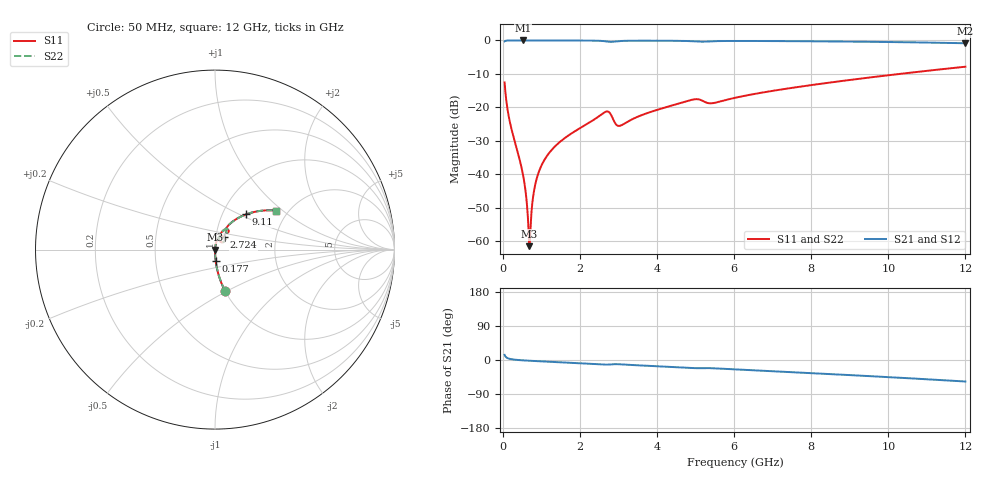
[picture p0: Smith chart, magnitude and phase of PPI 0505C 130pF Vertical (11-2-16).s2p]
# GHz S MA R 50
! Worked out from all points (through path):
!   1601 points, 50 MHz to 12 GHz, reference 50 ohm
!   highest |S21| = -0.01 dB at 528 MHz (marker M1); lowest = -0.8 dB at 12 GHz (marker M2)
!   group delay of S21, straight-line fit = 13.2 ps
!   lowest |S11| = -61.4 dB at 692.3 MHz (marker M3), VSWR 1.00, Z = 50.1 - j0.0122 ohm
!   |S11| at or under -10 dB: start of sweep to 10.29 GHz
!   |S22| runs from -61.4 to -7.8 dB; largest |S21 - S12| = 0
!   S11 on the Smith chart (normalised r, x): 50 MHz: 1.00, -0.49; 177 MHz: 1.00, -0.13; 2.724 GHz: 1.10, +0.16; 9.11 GHz: 1.29, +0.54; 12 GHz: 1.74, +0.91
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0.05  0.2362 -76.4  0.9714 13.5  0.9714 13.5  0.2362 -76.4
0.1769688  0.06444 -86.4  0.9974 3.2  0.9974 3.2  0.06444 -86.4
0.528  0.009816 -86.5  0.9992 -0.9  0.9992 -0.9  0.009816 -86.5
0.5952188  0.005517 -83.1  0.9992 -1.4  0.9992 -1.4  0.005517 -83.1
0.6549687  0.002217 -69.9  0.9991 -1.7  0.9991 -1.7  0.002217 -69.9
0.6923125  0.0008512 -8.2  0.9991 -1.9  0.9991 -1.9  0.0008512 -8.2
0.7296563  0.001972 61.8  0.9991 -2.2  0.9991 -2.2  0.001972 61.8
0.796875  0.005003 77.1  0.999 -2.5  0.999 -2.5  0.005003 77.1
0.856625  0.007599 80.1  0.999 -2.8  0.999 -2.8  0.007599 80.1
1.050812  0.01531 82.3  0.9988 -3.8  0.9988 -3.8  0.01531 82.3
1.416781  0.02829 81.9  0.9983 -5.6  0.9983 -5.6  0.02829 81.9
2.044156  0.05065 78.8  0.9964 -8.7  0.9964 -8.7  0.05065 78.8
2.723813  0.08708 54.0  0.9616 -12.2  0.9616 -12.2  0.08708 54.0
3.030031  0.05306 56.3  0.9784 -11.3  0.9784 -11.3  0.05306 56.3
4.038312  0.09327 70.3  0.9905 -16.7  0.9905 -16.7  0.09327 70.3
4.9495  0.1318 60.0  0.9714 -21.3  0.9714 -21.3  0.1318 60.0
5.405094  0.1153 56.6  0.9697 -21.6  0.9697 -21.6  0.1153 56.6
6.025  0.1393 62.0  0.9823 -24.8  0.9823 -24.8  0.1393 62.0
8.019156  0.2163 54.0  0.9712 -34.7  0.9712 -34.7  0.2163 54.0
9.109594  0.2618 48.6  0.9598 -40.4  0.9598 -40.4  0.2618 48.6
10.01331  0.3029 43.8  0.9474 -45.2  0.9474 -45.2  0.3029 43.8
12  0.4054 32.4  0.9076 -56.8  0.9076 -56.8  0.4054 32.4
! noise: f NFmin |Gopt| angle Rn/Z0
0.05  0.0003875  0.8639  0.2904  0.0006112
1.372  0.004125  0.6833  3.753  0.002521
2.701  0.0292  0.9007  7.572  0.06408
4.031  0.01409  0.7225  11.02  0.009982
5.36  0.038  0.8532  14.91  0.05432
6.682  0.01922  0.6746  17.87  0.01112
8.012  0.01977  0.6327  20.87  0.009802
9.341  0.02185  0.6187  23.89  0.01025
10.67  0.02453  0.6162  26.87  0.01129
12  0.02772  0.6208  29.83  0.01279
